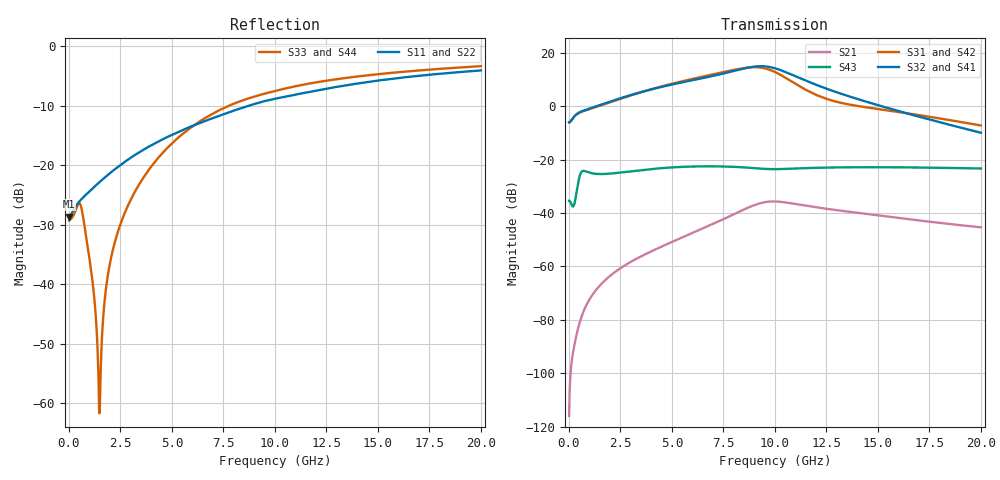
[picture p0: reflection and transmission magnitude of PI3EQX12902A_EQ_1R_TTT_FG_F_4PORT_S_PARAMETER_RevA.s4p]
! NPort=4 DATA=2000 NOISE=0 GROUPDELAY=0 COMPLEX_DATAFORMAT=POLAR
! NumOfBlock=1 NumOfParam=0
! .MODEL Smodel S TSTONEFILE=PI3EQX12902A_EQ_1R_TTT_FG_F_4PORT_S_PARAMETER_RevA.s4p TYPE=S
!  -- The above .MODEL line can be used for the S element in the netlist.
! The s parameter is extracted from the linear redriver, it is not bi-directional; only s(4,1)s(4,2) and s(3,1)s(3,2)
! should be the insertion loss
!Port definition:
!Port1 = input+
!Port2 = input-
!Port3 = output+
!Port4 = output-
# Hz S MA R  50
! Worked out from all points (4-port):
!   2000 points, 10 MHz to 20 GHz, reference 50 ohm
!   strongest paths, dB at 10 MHz, 5.01 GHz, 10.01 GHz, 15.01 GHz, 20 GHz:
!     S32: -6.0, 8.2, 14.2, 0.4, -9.9
!     S41: -6.0, 8.1, 14.1, 0.4, -9.9
!     S31: -6.0, 8.4, 12.8, -1.0, -7.2
!     S42: -6.0, 8.4, 12.7, -1.3, -7.3
!     S43: -35.3, -22.9, -23.5, -22.8, -23.3
!     S21: -116.0, -50.8, -35.7, -40.9, -45.3
!   lowest |S11| = -28.6 dB at 10 MHz (marker M1), VSWR 1.08, Z = 46.4 - j0.0607 ohm
!   |S11| at or under -10 dB: start of sweep to 8.729 GHz
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1e7  0.03704 -179.0  1.589e-06 51.9  0 0.0  0 0.0
     1.589e-06 51.9  0.03704 -179.0  0 0.0  0 0.0
     0.4991 1.1  0.4991 -178.9  0.03429 6.0  0.01709 -177.1
     0.4991 -178.9  0.4991 1.1  0.01709 -177.1  0.03429 6.0
5.91e9  0.2108 -111.9  0.004101 99.9  1.532e-06 -20.6  9.462e-07 87.5
        0.0041 99.9  0.2108 -111.9  9.493e-07 87.7  1.526e-06 -20.3
        3.194 -51.8  3.026 109.7  0.2065 -45.5  0.0739 145.7
        3.015 109.7  3.155 -52.3  0.07429 145.8  0.2059 -45.5
8.09e9  0.2906 -111.7  0.00984 76.7  7.821e-06 -84.4  4.733e-06 42.0
        0.009835 76.7  0.2906 -111.7  4.759e-06 42.0  7.793e-06 -84.1
        4.872 -111.2  4.664 50.7  0.3335 -66.9  0.07268 122.8
        4.637 50.6  4.798 -111.6  0.07315 122.7  0.3328 -66.8
9.31e9  0.3386 -113.6  0.01541 45.3  1.421e-05 -132.1  1.137e-05 -2.7
        0.01539 45.3  0.3386 -113.6  1.141e-05 -2.9  1.416e-05 -131.6
        5.311 -162.7  5.634 0.0  0.3908 -76.7  0.06759 113.4
        5.586 -0.0  5.227 -163.0  0.06798 113.2  0.3905 -76.6
1.044e10  0.3744 -115.9  0.016 8.9  1.551e-05 -171.4  1.667e-05 -55.8
          0.01596 8.9  0.3744 -115.8  1.667e-05 -56.0  1.548e-05 -170.8
          3.552 148.5  4.486 -52.5  0.4385 -84.0  0.06668 109.3
          4.439 -52.4  3.49 148.0  0.06697 109.0  0.4385 -83.9
1.244e10  0.437 -118.6  0.01215 -26.1  1.861e-05 160.6  1.909e-05 -121.3
          0.01213 -26.0  0.437 -118.6  1.902e-05 -121.4  1.87e-05 161.2
          1.404 117.1  2.181 -109.1  0.5106 -94.8  0.071 96.6
          2.159 -108.7  1.367 116.8  0.07103 96.3  0.5109 -94.7
2e10  0.6256 -131.7  0.005393 -76.6  3.966e-05 51.1  1.804e-05 95.6
      0.005417 -76.6  0.6256 -131.7  1.79e-05 96.1  3.998e-05 51.3
      0.4369 36.1  0.3192 128.9  0.6794 -119.6  0.06842 46.2
      0.3203 129.6  0.4309 36.9  0.06832 46.1  0.6797 -119.6
